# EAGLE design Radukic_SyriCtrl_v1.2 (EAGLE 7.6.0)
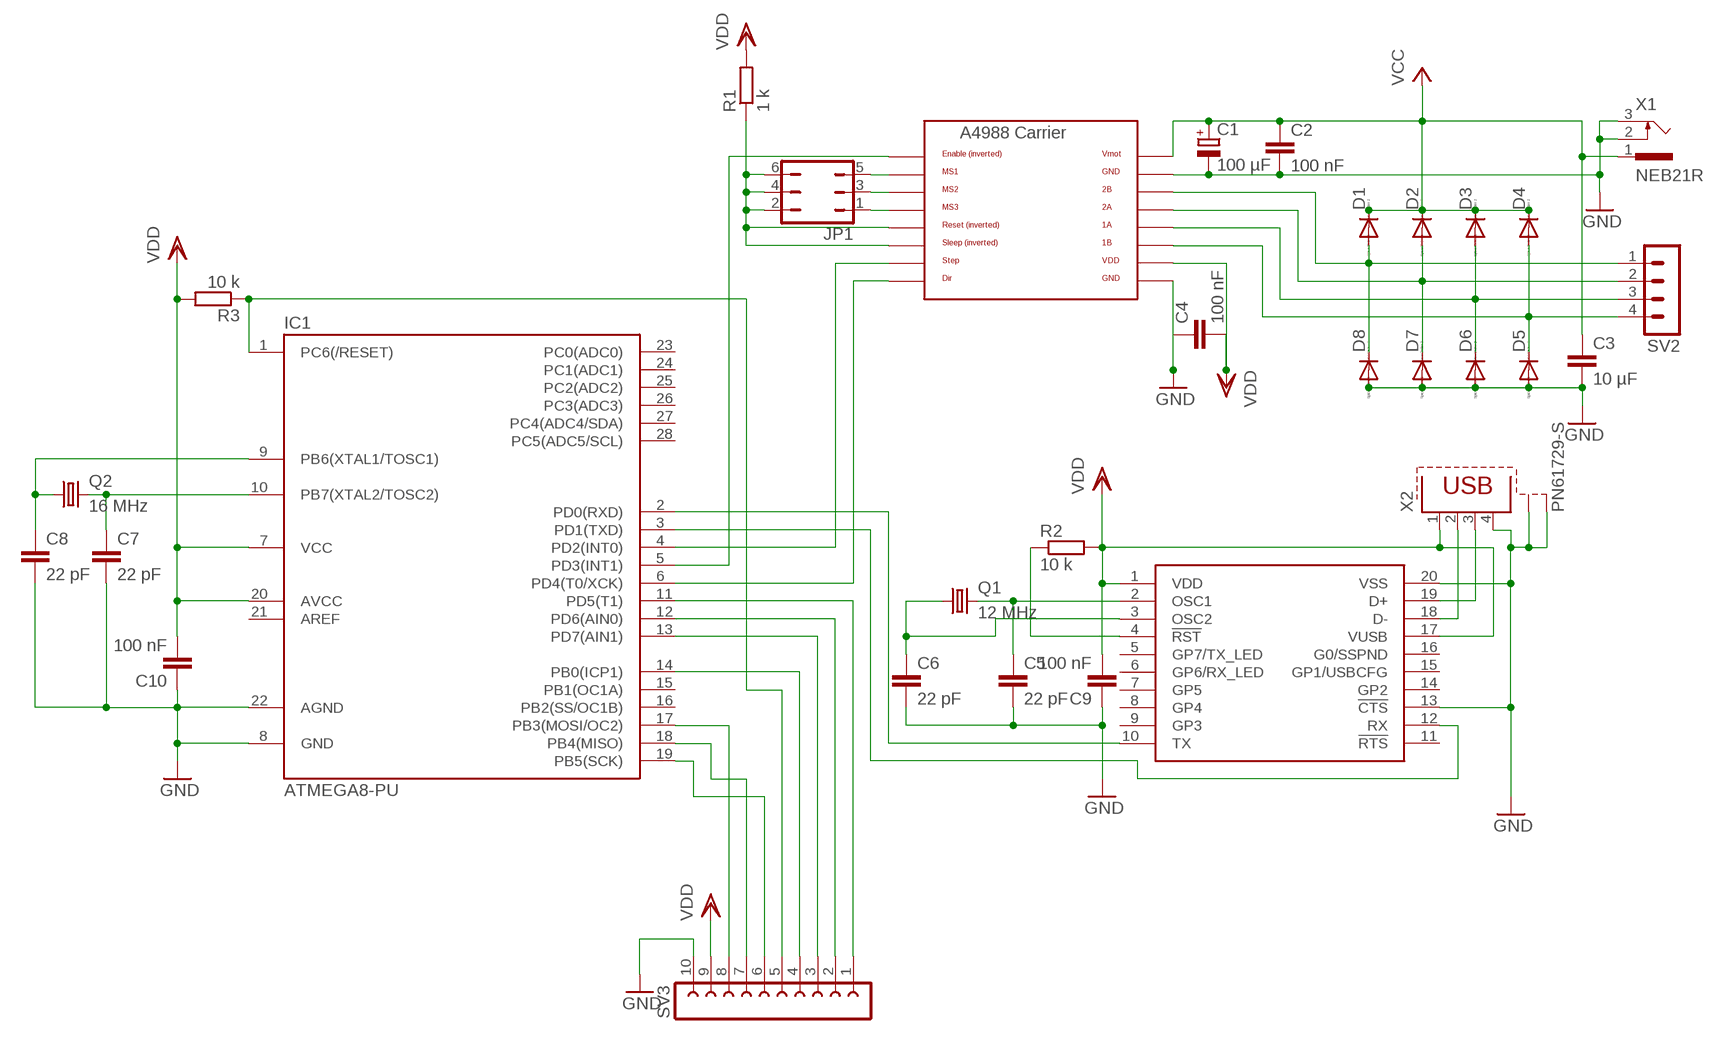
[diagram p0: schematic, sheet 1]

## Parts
C1  100 µF  CPOL-EUTAP5-80  [TAP5-80]
C2  100 nF  C-EU050-024X044  [C050-024X044]
C3  10 µF  C-EU075-032X103  [C075-032X103]
C4  100 nF  C-EU050-024X044  [C050-024X044]
C5  22 pF  C-EU050-024X044  [C050-024X044]
C6  22 pF  C-EU050-024X044  [C050-024X044]
C7  22 pF  C-EU050-024X044  [C050-024X044]
C8  22 pF  C-EU050-024X044  [C050-024X044]
C9  100 nF  C-EU050-024X044  [C050-024X044]
C10  100 nF  C-EU050-024X044  [C050-024X044]
D1  DIODE-D-2.5  [D-2.5]
D2  DIODE-D-2.5  [D-2.5]
D3  DIODE-D-2.5  [D-2.5]
D4  DIODE-D-2.5  [D-2.5]
D5  DIODE-D-2.5  [D-2.5]
D6  DIODE-D-2.5  [D-2.5]
D7  DIODE-D-2.5  [D-2.5]
D8  DIODE-D-2.5  [D-2.5]
IC  POLOLU_A4983CARRIER  [A4988BREAKOUT]
IC1  ATMEGA8-PU  [DIL28-3]
JP1  JP3Q  [JP3Q]
Q1  12 MHz  CRYSTALHC49S  [HC49/S]
Q2  16 MHz  CRYSTALHC49S  [HC49/S]
R1  1 k  R-EU_VMTA55  [VMTA55]
R2  10 k  R-EU_VMTA55  [VMTA55]
R3  10 k  R-EU_VMTA55  [VMTA55]
SV2  MA04-1  [MA04-1]
SV3  FE10-1  [FE10]
U$2  MCP2200SOIC  [MCP2200]
X1  NEB21R  [NEB21R]
X2  PN61729-S  [PN61729-S]

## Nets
GND: C1.- C2.2 C3.2 C4.1 C5.2 C6.2 C7.2 C8.2 C9.1 C10.1 D5.A D6.A D7.A D8.A IC1.8(GND) IC1.22(AGND) IC.GND IC.GND@0(GND) SV3.10 U$2.13(!CTS) U$2.20(VSS) X1.2 X1.3 X2.4 X2.S1 X2.S2
N$1: U$2.18(D-) X2.2
N$2: IC.MS1 JP1.5
N$3: D1.A D8.C IC.2B SV2.1
N$4: D2.A D7.C IC.2A SV2.2
N$5: D3.A D6.C IC.1A SV2.3
N$6: D4.A D5.C IC.1B SV2.4
N$7: IC.MS2 JP1.3
N$8: IC.MS3 JP1.1
N$9: IC1.6(PD4(T0/XCK)) IC.DIR
N$10: IC1.5(PD3(INT1)) IC.EN
N$11: IC1.4(PD2(INT0)) IC.STEP
N$12: IC1.11(PD5(T1)) SV3.1
N$13: IC1.12(PD6(AIN0)) SV3.2
N$14: IC1.13(PD7(AIN1)) SV3.3
N$15: IC1.2(PD0(RXD)) U$2.10(TX)
N$16: U$2.19(D+) X2.3
N$17: IC1.17(PB3(MOSI/OC2)) SV3.8
N$18: IC1.3(PD1(TXD)) U$2.12(RX)
N$19: C5.1 Q1.2 U$2.2(OSC1)
N$20: C6.1 Q1.1 U$2.3(OSC2)
N$21: IC1.18(PB4(MISO)) SV3.7
N$22: R2.1 U$2.4(!RST)
N$23: IC1.1(PC6(/RESET)) R3.1 SV3.5
N$24: IC.RST IC.SLP(SLEEP) JP1.2 JP1.4 JP1.6 R1.1
N$25: IC1.19(PB5(SCK)) SV3.6
N$26: IC1.14(PB0(ICP1)) SV3.4
N$27: C7.1 IC1.10(PB7(XTAL2/TOSC2)) Q2.2
N$29: C8.1 IC1.9(PB6(XTAL1/TOSC1)) Q2.1
VCC: C1.+ C2.1 C3.1 D1.C D2.C D3.C D4.C IC.VMOT X1.1
VDD: C4.2 C9.2 C10.2 IC1.7(VCC) IC1.20(AVCC) IC.VDD R1.2 R2.2 R3.2 SV3.9 U$2.1(VDD) U$2.17(VUSB) X2.1
Unconnected: IC1.15(PB1(OC1A)) IC1.16(PB2(SS/OC1B)) IC1.21(AREF) IC1.23(PC0(ADC0)) IC1.24(PC1(ADC1)) IC1.25(PC2(ADC2)) IC1.26(PC3(ADC3)) IC1.27(PC4(ADC4/SDA)) IC1.28(PC5(ADC5/SCL)) U$2.5(GP7/TX_LED) U$2.6(GP6/RX_LED) U$2.7(GP5) U$2.8(GP4) U$2.9(GP3) U$2.11(!RTS) U$2.14(GP2) U$2.15(GP1/USBCFG) U$2.16(G0/SSPND)

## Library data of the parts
C1 = resistor:CPOL-EU: POLARIZED CAPACITOR, European symbol
C2-C10 = resistor:C-EU: CAPACITOR, European symbol
D1-D8 = diode:DIODE-: DIODE
IC = RepRapjr:POLOLU_A4983CARRIER
IC1 = atmega8:ATMEGA8-PU
JP1 = jumper:JP3Q: JUMPER
Q1 Q2 = crystal:CRYSTAL: CRYSTAL; OC_FARNELL: 1667008; OC_NEWARK: unknown
R1-R3 = resistor:R-EU_: RESISTOR, European symbol
SV2 = con-lstb:MA04-1: PIN HEADER; OC_FARNELL: unknown; OC_NEWARK: unknown
SV3 = con-lsta:FE10-1: FEMALE HEADER; OC_FARNELL: unknown; OC_NEWARK: unknown
U$2 = mcp2200:MCP2200: USB to serial converter by micreochip
X1 = con-lumberg:NEB21R: Netzgeräte-Einbaukupplung abgewinkelte Ausführung mit Öffner Source: http://www.lumberg.com/Produkte/PDFs/NEB21R.pdf; MPN: NEB 21 R; OC_FARNELL: 1217037; OC_NEWARK: 97K6458
X2 = con-berg:PN61729-S: BERG USB connector; OC_FARNELL: unknown; OC_NEWARK: unknown

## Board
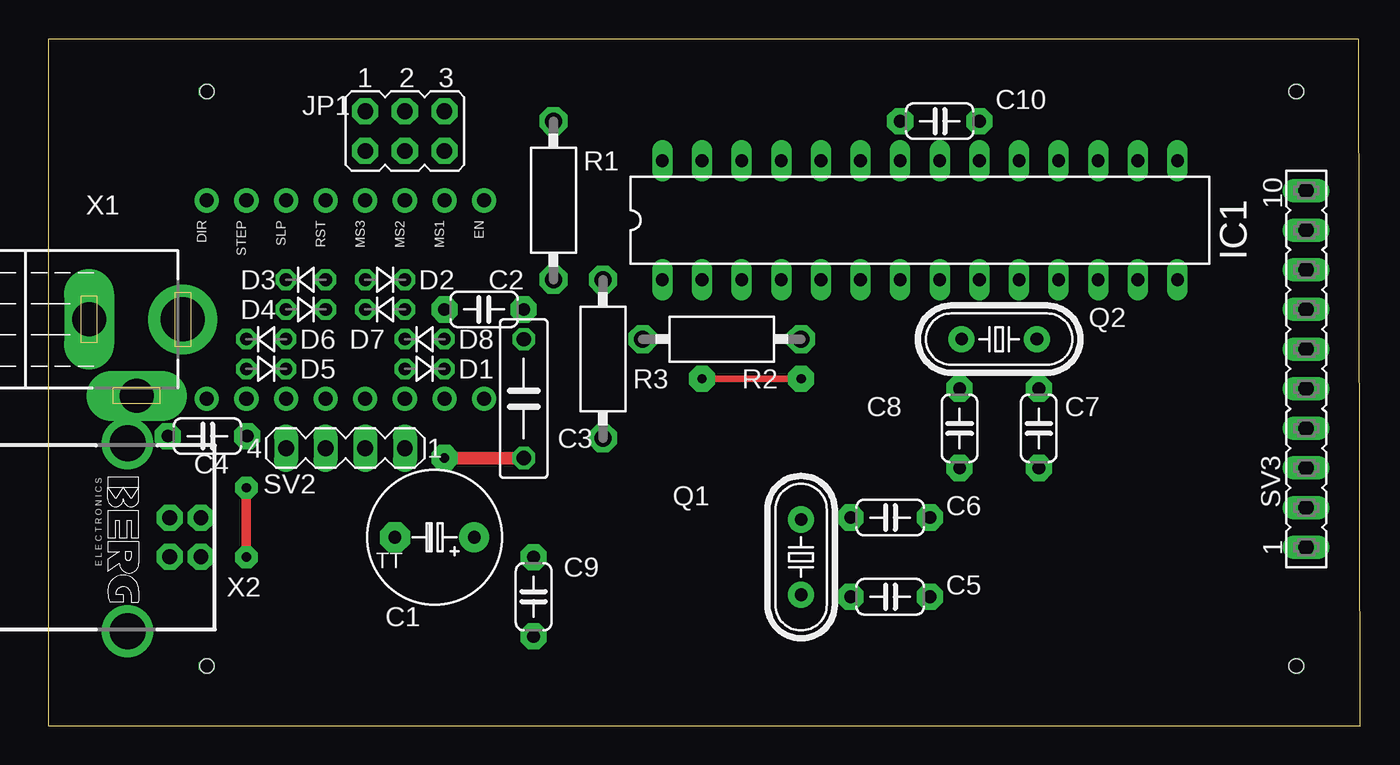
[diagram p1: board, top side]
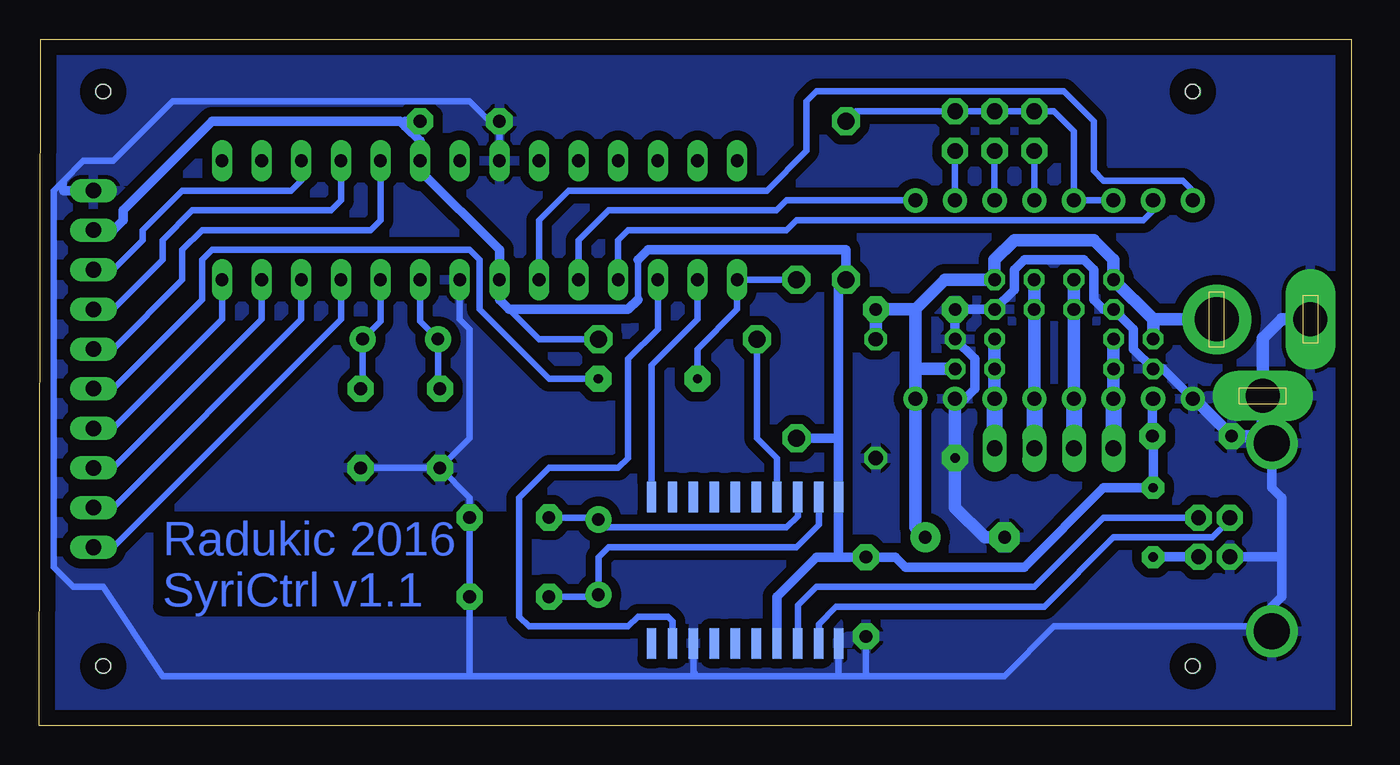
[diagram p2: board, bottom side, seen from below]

Size 84.12 x 44 mm. Coordinates in mm from the lower left corner, seen from the top.
Outline: 0,0 84.12,0 84,44 0,44 0,0
Copper layers (1*16): Top 0.035mm / dielectric 1.5mm / Bottom 0.035mm
Design rules "default": minimum track width 10mil, minimum drill 24mil, track to track 8mil, track to pad 8mil, pad to pad 8mil, via to via 8mil, smd to smd 8mil, copper to edge 40mil, drill to drill 8mil, minimum pad ring 10mil, minimum via ring 8mil, stop-mask expansion 4mil, vias tented up to drill 0mil, thermal gap 10mil
Holes 0.9 mm at 10.16,3.81 10.16,40.64 80.01,3.81 80.01,40.64

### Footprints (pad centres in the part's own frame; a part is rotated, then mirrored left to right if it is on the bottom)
TAP5-80 = drill 0.813 pad 1.93: + -2.54,0 | drill 0.813 pad 1.93 octagon: - 2.54,0
C050-024X044 = drill 0.813 pad 1.676 octagon: 1 -2.54,0; 2 2.54,0
C075-032X103 = drill 0.914 octagon: 1 -3.81,0; 2 3.81,0
D-2.5 = drill 0.813 octagon: A 1.27,0; C -1.27,0
A4988BREAKOUT = drill 0.9 pad 1.549: 1A 8.89,1.27; 1B 11.43,1.27; 2A 6.35,1.27; 2B 3.81,1.27; DIR 16.51,-11.43; EN -1.27,-11.43; GND 16.51,1.27; GND@0 1.27,1.27; MS1 1.27,-11.43; MS2 3.81,-11.43; MS3 6.35,-11.43; RST 8.89,-11.43; SLP 11.43,-11.43; STEP 13.97,-11.43; VDD 13.97,1.27; VMOT -1.27,1.27
DIL28-3 = drill 0.813 long: 1 -16.51,-3.81; 2 -13.97,-3.81; 3 -11.43,-3.81; 4 -8.89,-3.81; 5 -6.35,-3.81; 6 -3.81,-3.81; 7 -1.27,-3.81; 8 1.27,-3.81; 9 3.81,-3.81; 10 6.35,-3.81; 11 8.89,-3.81; 12 11.43,-3.81; 13 13.97,-3.81; 14 16.51,-3.81; 15 16.51,3.81; 16 13.97,3.81; 17 11.43,3.81; 18 8.89,3.81; 19 6.35,3.81; 20 3.81,3.81; 21 1.27,3.81; 22 -1.27,3.81; 23 -3.81,3.81; 24 -6.35,3.81; 25 -8.89,3.81; 26 -11.43,3.81; 27 -13.97,3.81; 28 -16.51,3.81
JP3Q = drill 1 pad 1.676 octagon: 1 -2.54,-1.27; 2 -2.54,1.27; 3 0,-1.27; 4 0,1.27; 5 2.54,-1.27; 6 2.54,1.27
HC49/S = drill 0.813 pad 1.676: 1 -2.413,0; 2 2.413,0
VMTA55 = drill 1.1 pad 1.778 octagon: 1 -5.08,0; 2 5.08,0
MA04-1 = drill 1.016 long: 1 -3.81,0; 2 -1.27,0; 3 1.27,0; 4 3.81,0
FE10 = drill 1 long: 1 -11.43,0; 2 -8.89,0; 3 -6.35,0; 4 -3.81,0; 5 -1.27,0; 6 1.27,0; 7 3.81,0; 8 6.35,0; 9 8.89,0; 10 11.43,0
MCP2200 = smd 0.6 x 1.95: 1 -0.6,0.145; 2 0.67,0.145; 3 2.01,0.145; 4 3.35,0.145; 5 4.69,0.145; 6 6.03,0.145; 7 7.37,0.145; 8 8.71,0.145; 9 10.05,0.145; 10 11.39,0.145; 11 11.39,9.525; 12 10.05,9.525; 13 8.71,9.525; 14 7.37,9.525; 15 6.03,9.525; 16 4.69,9.525; 17 3.35,9.525; 18 2.01,9.525; 19 0.67,9.525; 20 -0.6,9.525
NEB21R = drill 2.8 pad 4.445: 1 0,7.35 | drill 2.2 pad 2.54 long: 2 4.9,4.4; 3 0,1.35
PN61729-S = drill 0.95 pad 1.676 octagon: 1 1.25,4.71; 2 -1.25,4.71; 3 -1.25,2.71; 4 1.25,2.71 | drill 2.3 pad 2.9: S1 -6.02,0; S2 6.02,0

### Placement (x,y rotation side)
C1  24.77,12.06 180 top
C2  27.94,26.67 180 top
C3  30.48,20.95 270 top
C4  10.2,18.55 0 top
C5  53.98,8.26 0 top
C6  53.98,13.34 0 top
C7  63.5,19.05 270 top
C8  58.42,19.05 270 top
C9  31.11,8.26 90 top
C10  57.15,38.73 0 top
D1  24.13,22.86 180 top
D2  21.59,28.57 180 top
D3  16.51,28.57 0 top
D4  13.97,24.77 0 top
D5  13.97,22.86 180 top
D6  16.51,26.67 180 top
D7  21.59,26.67 0 top
D8  24.13,24.77 0 top
IC  26.67,22.23 180 top
IC1  55.88,32.38 0 top
JP1  22.86,38.1 0 top
Q1  48.26,10.79 270 top
Q2  60.96,24.77 0 top
R1  32.38,33.66 270 top
R2  43.18,24.77 0 top
R3  35.56,23.5 270 top
SV2  19.05,17.78 180 top
SV3  80.64,22.86 90 top
U$2  33.46,14.8 180 bottom
X1  1.27,26.04 270 top
X2  5.08,12.06 270 top

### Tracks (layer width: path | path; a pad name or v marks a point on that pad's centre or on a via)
GND  (via drill 0.6 pad 0.61, 0.6 pad 1.68)
  Top 0.813: v25.4,17.14 C3.2
  Bottom 0.406: 31.11,3.17 22.23,3.17 19.05,6.35 5.38,6.35 X2.S2 | 31.11,3.17 33.02,3.17 | 33.02,3.17 41.91,3.17 | U$2.13 42.17,3.44 41.91,3.17 | U$2.20 32.86,3.33 33.02,3.17 | 41.91,3.17 56.52,3.17 | 56.52,3.17 C5.2 C6.2 56.52,14.61 C8.2 | C8.2 C7.2 | C8.2 56.52,18.41 56.52,25.4 57.15,26.04 IC1.8 | 82.55,34.29 82.55,34.92 | 55.24,38.73 56.52,40.01 75.56,40.01 79.38,36.2 81.28,36.2 82.55,34.92 | 55.24,38.73 54.61,38.1 IC1.22 | 56.52,3.17 76.2,3.17 80.01,8.89 81.92,8.89 83.19,10.16 83.19,34.29 82.55,34.92 | C9.1 31.11,3.17 | C10.1 55.24,38.73 | 4.45,10.81 4.45,10.79
  Bottom 0.61: SV3.10 82.55,34.29 | X2.S1 v5.08,18.03 5.08,15.24 4.45,14.61 4.45,10.79 | 4.45,10.79 4.45,8.26 5.08,7.62 v5.08,6.1 X2.S2 | IC.GND@0 24.77,20.95 24.13,21.59 24.13,23.5 D8.A C2.2 D7.A 21.59,27.94 21.59,29.21 20.95,29.84 17.14,29.84 16.51,29.21 16.51,27.3 15.88,26.67 D6.A 13.97,25.4 13.97,24.13 D5.A 12.06,22.86 IC.GND | X2.4 4.46,10.81 4.45,10.79
  Bottom 0.813: IC.GND 10.07,20.95 C4.1 5.54,18.55 X2.S1 | X1.3 4.45,26.04 5.67,24.81 X1.2 5.67,18.62 v5.08,18.03 | C1.- 23.5,12.06 25.4,13.97 v25.4,17.14 IC.GND@0
  pour Bottom (isolate 0.61): -0.64,44.45 -0.64,-0.64 85.09,-0.64 85.09,44.45
N$1
  Bottom 0.406: X2.2 15.89,13.31 20.32,8.89 34.29,8.89 35.47,7.71 U$2.18
N$2
  Bottom 0.406: JP1.5 IC.MS1
N$3
  Bottom 0.813: D8.C D1.A IC.2B
  Bottom 1.016: IC.2B SV2.1
N$4
  Bottom 0.813: IC.2A D7.C D2.A
  Bottom 1.016: IC.2A SV2.2
N$5
  Bottom 0.813: IC.1A D6.C D3.A
  Bottom 1.016: IC.1A SV2.3
N$6
  Bottom 0.813: IC.1B D5.C D4.A
  Bottom 1.016: IC.1B SV2.4
N$7
  Bottom 0.406: JP1.3 IC.MS2
N$8
  Bottom 0.406: JP1.1 IC.MS3
N$9
  Bottom 0.406: IC.DIR 10.16,34.29 10.79,34.92 15.88,34.92 16.51,35.56 16.51,38.73 18.41,40.64 34.29,40.64 34.92,40.01 34.92,36.83 37.47,34.29 50.16,34.29 52.07,32.38 IC1.6
N$10
  Bottom 0.406: IC.EN 36.2,33.66 36.83,33.02 47.62,33.02 49.53,31.11 IC1.5
N$11
  Bottom 0.406: IC.STEP 12.7,33.02 13.34,32.38 35.56,32.38 36.2,31.75 46.35,31.75 46.99,31.11 IC1.4
N$12
  Bottom 0.406: SV3.1 79.38,11.43 64.77,26.04 IC1.11
N$13
  Bottom 0.406: SV3.2 79.38,13.97 67.31,26.04 IC1.12
N$14
  Bottom 0.406: SV3.3 79.38,16.51 69.85,26.04 IC1.13
N$15
  Bottom 0.406: U$2.10 44.85,23.09 41.91,26.04 IC1.2
N$16
  Bottom 0.406: X2.3 7.79,13.16 8.89,12.06 15.24,12.06 19.68,7.62 33.02,7.62 34.13,6.5 U$2.19
N$17
  Bottom 0.406: IC1.17 67.31,34.92 67.94,34.29 74.93,34.29 77.47,31.75 77.47,31.11 79.38,29.21 SV3.8
N$18
  Bottom 0.406: U$2.12 43.51,6.68 43.81,6.99 45.72,6.99 46.35,6.35 52.7,6.35 53.34,6.99 53.34,14.61 51.44,16.51 46.99,16.51 46.35,17.14 46.35,23.5 44.45,25.4 IC1.3
N$19
  Bottom 0.406: U$2.2 34.13,12.86 35.56,11.43 47.62,11.43 48.26,10.79 Q1.2 48.39,8.26 C5.1
N$20
  Bottom 0.406: U$2.3 35.47,13.42 36.2,12.7 47.75,12.7 Q1.1 48.39,13.34 C6.1
N$21
  Bottom 0.406: IC1.18 64.77,33.66 65.41,33.02 74.3,33.02 76.2,31.11 76.2,29.84 79.38,26.67 SV3.7
N$22
  Bottom 0.406: U$2.4 36.81,17.13 38.1,18.41 R2.1
N$23  (via drill 0.6 pad 1.68)
  Top 0.406: v41.91,22.23 v48.26,22.23
  Bottom 0.406: R3.1 IC1.1 39.37,26.67 41.91,24.13 v41.91,22.23 | v48.26,22.23 51.44,22.23 55.88,26.67 55.88,29.84 56.52,30.48 73.03,30.48 73.66,29.84 73.66,27.3 79.38,21.59 SV3.5
N$24
  Bottom 0.406: IC.SLP IC.RST 17.78,38.1 19.05,39.37 JP1.2 JP1.4 JP1.6 31.75,39.37 R1.1
N$25
  Bottom 0.406: IC1.19 62.23,32.38 62.87,31.75 73.66,31.75 74.93,30.48 74.93,28.57 79.38,24.13 SV3.6
N$26
  Bottom 0.406: SV3.4 79.38,19.05 72.39,26.04 IC1.14
N$27
  Bottom 0.406: IC1.10 62.23,25.91 Q2.2 63.37,21.72 C7.1
N$28  (via drill 0.6 pad 0.61)
  other vias: 10.16,40.64
N$29
  Bottom 0.406: IC1.9 59.69,25.91 Q2.1 58.55,21.72 C8.1
N$30  (via drill 0.6 pad 0.61)
  other vias: 10.16,3.81
N$31  (via drill 0.6 pad 0.61)
  other vias: 80.01,3.81
N$32  (via drill 0.6 pad 0.61)
  other vias: 80.01,40.64
VCC
  Bottom 0.813: D4.C 12.7,26.04 | 12.7,26.04 D3.C 15.24,29.84 16.51,31.11 21.59,31.11 22.86,29.84 D2.C 26.04,28.57 27.94,26.67 | 27.94,26.67 27.94,22.86 | 27.94,22.86 IC.VMOT 27.94,12.7 C1.+ | 27.94,26.67 C2.1 C3.1 | D1.C 27.94,22.86 | X1.1 12.7,26.04
VDD  (via drill 0.6 pad 1.42)
  Top 0.61: v12.7,10.79 v12.7,15.24
  Bottom 0.406: 45.72,27.3 45.72,29.84 | R2.2 52.07,24.77 53.98,26.67
  Bottom 0.61: R3.2 33.02,18.41 | 33.02,18.41 32.86,18.41 32.86,28.73 R1.2 32.38,30.48 45.09,30.48 45.72,29.84 | 45.72,27.3 46.35,26.67 53.98,26.67 54.61,27.3 IC1.7 54.61,30.48 59.69,35.56 IC1.20 59.69,37.47 60.64,38.42 | SV3.9 79.38,31.75 78.74,32.38 78.74,33.02 73.03,38.73 60.96,38.73 60.64,38.42 | C10.2 60.64,38.73 60.64,38.42 | IC.VDD 12.74,20.91 C4.2 12.7,17.87 v12.7,15.24 15.88,15.24 20.95,10.16 28.57,10.16 29.21,10.79 C9.2 33.02,10.79 | 33.02,10.79 34.29,10.79 36.81,8.27 U$2.17 | 33.02,10.79 32.86,10.95 U$2.1 32.86,18.26 33.02,18.41 | X2.1 12.68,10.81 v12.7,10.79

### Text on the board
Bottom: Radukic 2016 / SyriCtrl v1.1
